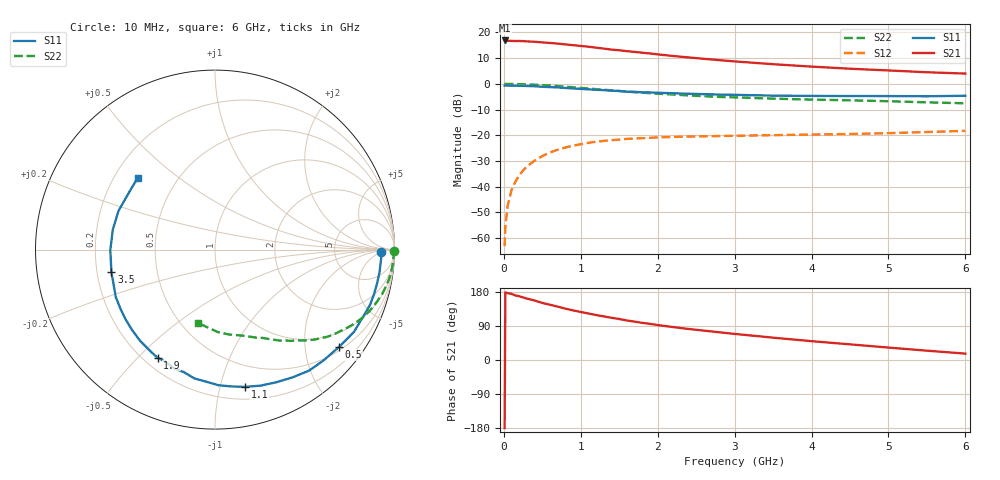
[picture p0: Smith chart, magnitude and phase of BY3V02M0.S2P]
! SIEMENS Small Signal Semiconductors
! BFY420
! Si NPN RF SIEGET Grounded Emitter Transistor in MICRO-X
! VCE = 3 V  IC = 2 mA
! Common Emitter S-Parameters:  October  1996
# GHz  S  MA  R  50
!  f  S11  S21  S12  S22
! GHz  MAG  ANG  MAG  ANG  MAG  ANG  MAG  ANG
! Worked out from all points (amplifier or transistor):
!   36 points, 10 MHz to 6 GHz, reference 50 ohm
!   highest |S21| = 16.9 dB at 10 MHz (marker M1)
!   |S21| within 3 dB of that: start of sweep to 1.253 GHz
!   unconditionally stable (mu >= 1): 4.005 GHz to end of sweep
!   at 250 MHz: K = 0.06, MSG = 25.1 dB, |S12| = -33.6 dB
!   at 1.4 GHz: K = 0.29, MSG = 17.6 dB, |S12| = -21.9 dB
!   at 6 GHz: K = 1.25, MAG = 8.1 dB, |S12| = -18.3 dB
!   S11 on the Smith chart (normalised r, x): 10 MHz: 25, -5; 500 MHz: 0.59, -2.79; 1.1 GHz: 0.30, -1.20; 1.9 GHz: 0.25, -0.57; 3.5 GHz: 0.26, -0.10; 6 GHz: 0.30, +0.36
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0.01  0.9269 -0.8  6.983 -179.6  0.0007 76.9  0.997 -0.3
0.02  0.9285 -1.5  6.963 178.3  0.0017 75.0  0.999 -0.7
0.05  0.9263 -3.9  6.855 176.4  0.0043 84.2  0.9958 -1.9
0.1  0.9253 -8.0  6.85 174.4  0.0086 87.0  0.9947 -3.8
0.15  0.9223 -11.7  6.799 170.4  0.0125 81.3  0.9916 -5.7
0.2  0.9203 -15.6  6.807 168.3  0.0167 80.1  0.9889 -7.4
0.25  0.9174 -19.4  6.78 165.0  0.0208 78.3  0.9839 -9.4
0.4  0.8998 -30.7  6.592 157.0  0.0322 72.5  0.9639 -14.8
0.5  0.8785 -38.1  6.402 150.6  0.0395 68.4  0.9461 -18.2
0.7  0.8542 -52.1  6.074 140.8  0.0524 60.7  0.9057 -24.7
0.8  0.8325 -58.8  5.852 135.6  0.0579 56.9  0.8817 -27.7
0.9  0.8142 -65.2  5.648 130.8  0.0631 53.7  0.8586 -30.3
1.1  0.7827 -77.7  5.281 122.7  0.0715 47.5  0.8123 -35.6
1.4  0.7369 -94.0  4.633 111.4  0.0804 40.4  0.7501 -41.9
1.6  0.7043 -104.3  4.318 104.3  0.0852 36.2  0.7085 -45.6
1.9  0.682 -118.0  3.899 95.4  0.0895 31.1  0.6593 -50.5
2.2  0.6574 -129.4  3.483 86.9  0.0931 27.1  0.6221 -54.6
2.8  0.62 -148.7  2.896 73.1  0.0969 22.0  0.5574 -61.9
3.5  0.5905 -167.8  2.413 58.9  0.1007 18.3  0.5165 -69.3
4.5  0.5801 169.0  1.97 41.3  0.1061 15.9  0.479 -80.7
5.5  0.5748 147.1  1.682 24.6  0.1159 14.6  0.4375 -94.7
6  0.5875 137.3  1.585 16.8  0.1221 13.9  0.4189 -102.7
